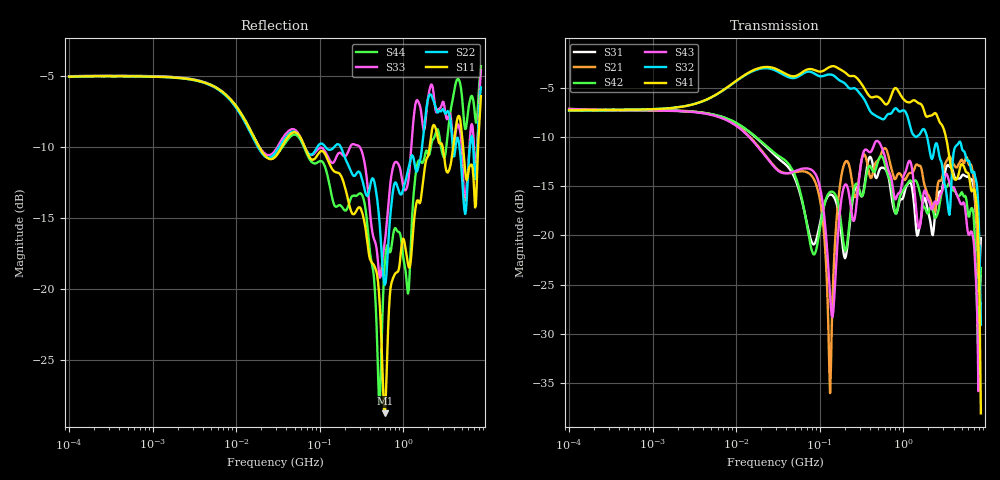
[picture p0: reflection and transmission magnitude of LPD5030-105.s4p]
# MHz S MA R 50
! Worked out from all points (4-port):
!   498 points, 100 kHz to 8.5 GHz, reference 50 ohm
!   strongest paths, dB at 100 kHz, 1.698 MHz, 29.49 MHz, 500.7 MHz, 8.5 GHz:
!     S41: -7.3, -7.1, -3.1, -5.9, -38.1
!     S32: -7.3, -7.1, -3.3, -8.0, -29.1
!     S43: -7.2, -7.4, -13.2, -10.5, -26.9
!     S42: -7.3, -7.3, -11.7, -12.4, -23.3
!     S21: -7.2, -7.3, -13.1, -12.4, -24.1
!     S31: -7.3, -7.3, -11.9, -13.7, -20.3
!   lowest |S11| = -28.7 dB at 601 MHz (marker M1), VSWR 1.08, Z = 50.8 - j3.62 ohm
!   |S11| at or under -10 dB: 66.13 MHz to 2.071 GHz (2.005 GHz wide, 188 % of centre); 2.959 GHz to 3.965 GHz (1.007 GHz wide, 29.1 % of centre); 5.211 GHz to 7.874 GHz (2.663 GHz wide, 40.7 % of centre)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
0.1  0.5584 3.5  0.4389 -5.5  0.4298 -175.5  0.4316 5.5
     0.4389 -5.5  0.5582 3.6  0.431 5.4  0.4305 -175.6
     0.4298 -175.5  0.431 5.4  0.5592 3.6  0.4377 -5.6
     0.4316 5.5  0.4305 -175.6  0.4377 -5.6  0.5599 3.7
76.95543  0.2887 -29.1  0.2041 67.7  0.09735 -112.9  0.6989 -11.2
          0.2041 67.7  0.2972 -18.4  0.677 -15.8  0.09089 -110.0
          0.09735 -112.9  0.677 -15.8  0.2964 -19.6  0.2168 66.8
          0.6989 -11.2  0.09089 -110.0  0.2168 66.8  0.2839 -33.1
133.1311  0.2729 -43.0  0.01582 42.4  0.1611 64.2  0.7173 -22.1
          0.01582 42.4  0.3087 -25.9  0.6555 -28.8  0.166 59.2
          0.1611 64.2  0.6555 -28.8  0.2829 -26.4  0.04928 -0.9
          0.7173 -22.1  0.166 59.2  0.04928 -0.9  0.2274 -50.0
191.855  0.2387 -56.6  0.2229 49.2  0.08264 17.2  0.6811 -37.9
         0.2229 49.2  0.3001 -41.7  0.598 -42.8  0.09254 10.6
         0.08264 17.2  0.598 -42.8  0.2941 -31.0  0.1724 41.2
         0.6811 -37.9  0.09254 10.6  0.1724 41.2  0.1916 -45.8
601.0223  0.03669 -76.2  0.2773 -63.6  0.2182 -73.3  0.4657 -92.0
          0.2773 -63.6  0.1036 -74.8  0.3929 -92.0  0.2309 -79.4
          0.2182 -73.3  0.3929 -92.0  0.1466 -48.1  0.2527 -83.3
          0.4657 -92.0  0.2309 -79.4  0.2527 -83.3  0.1226 -5.8
4588.001  0.4065 -179.2  0.2288 138.6  0.1942 124.5  0.2034 103.5
          0.2288 138.6  0.3328 164.6  0.2934 117.7  0.1582 113.3
          0.1942 124.5  0.2934 117.7  0.3777 171.9  0.1535 119.1
          0.2034 103.5  0.1582 113.3  0.1535 119.1  0.5464 -179.9
8500  0.4766 -33.1  0.06231 -8.2  0.09675 -0.8  0.01249 -62.6
      0.06231 -8.2  0.5115 -38.9  0.03519 -158.0  0.06831 22.4
      0.09675 -0.8  0.03519 -158.0  0.5868 -31.7  0.04518 22.6
      0.01249 -62.6  0.06831 22.4  0.04518 22.6  0.6074 -32.4
